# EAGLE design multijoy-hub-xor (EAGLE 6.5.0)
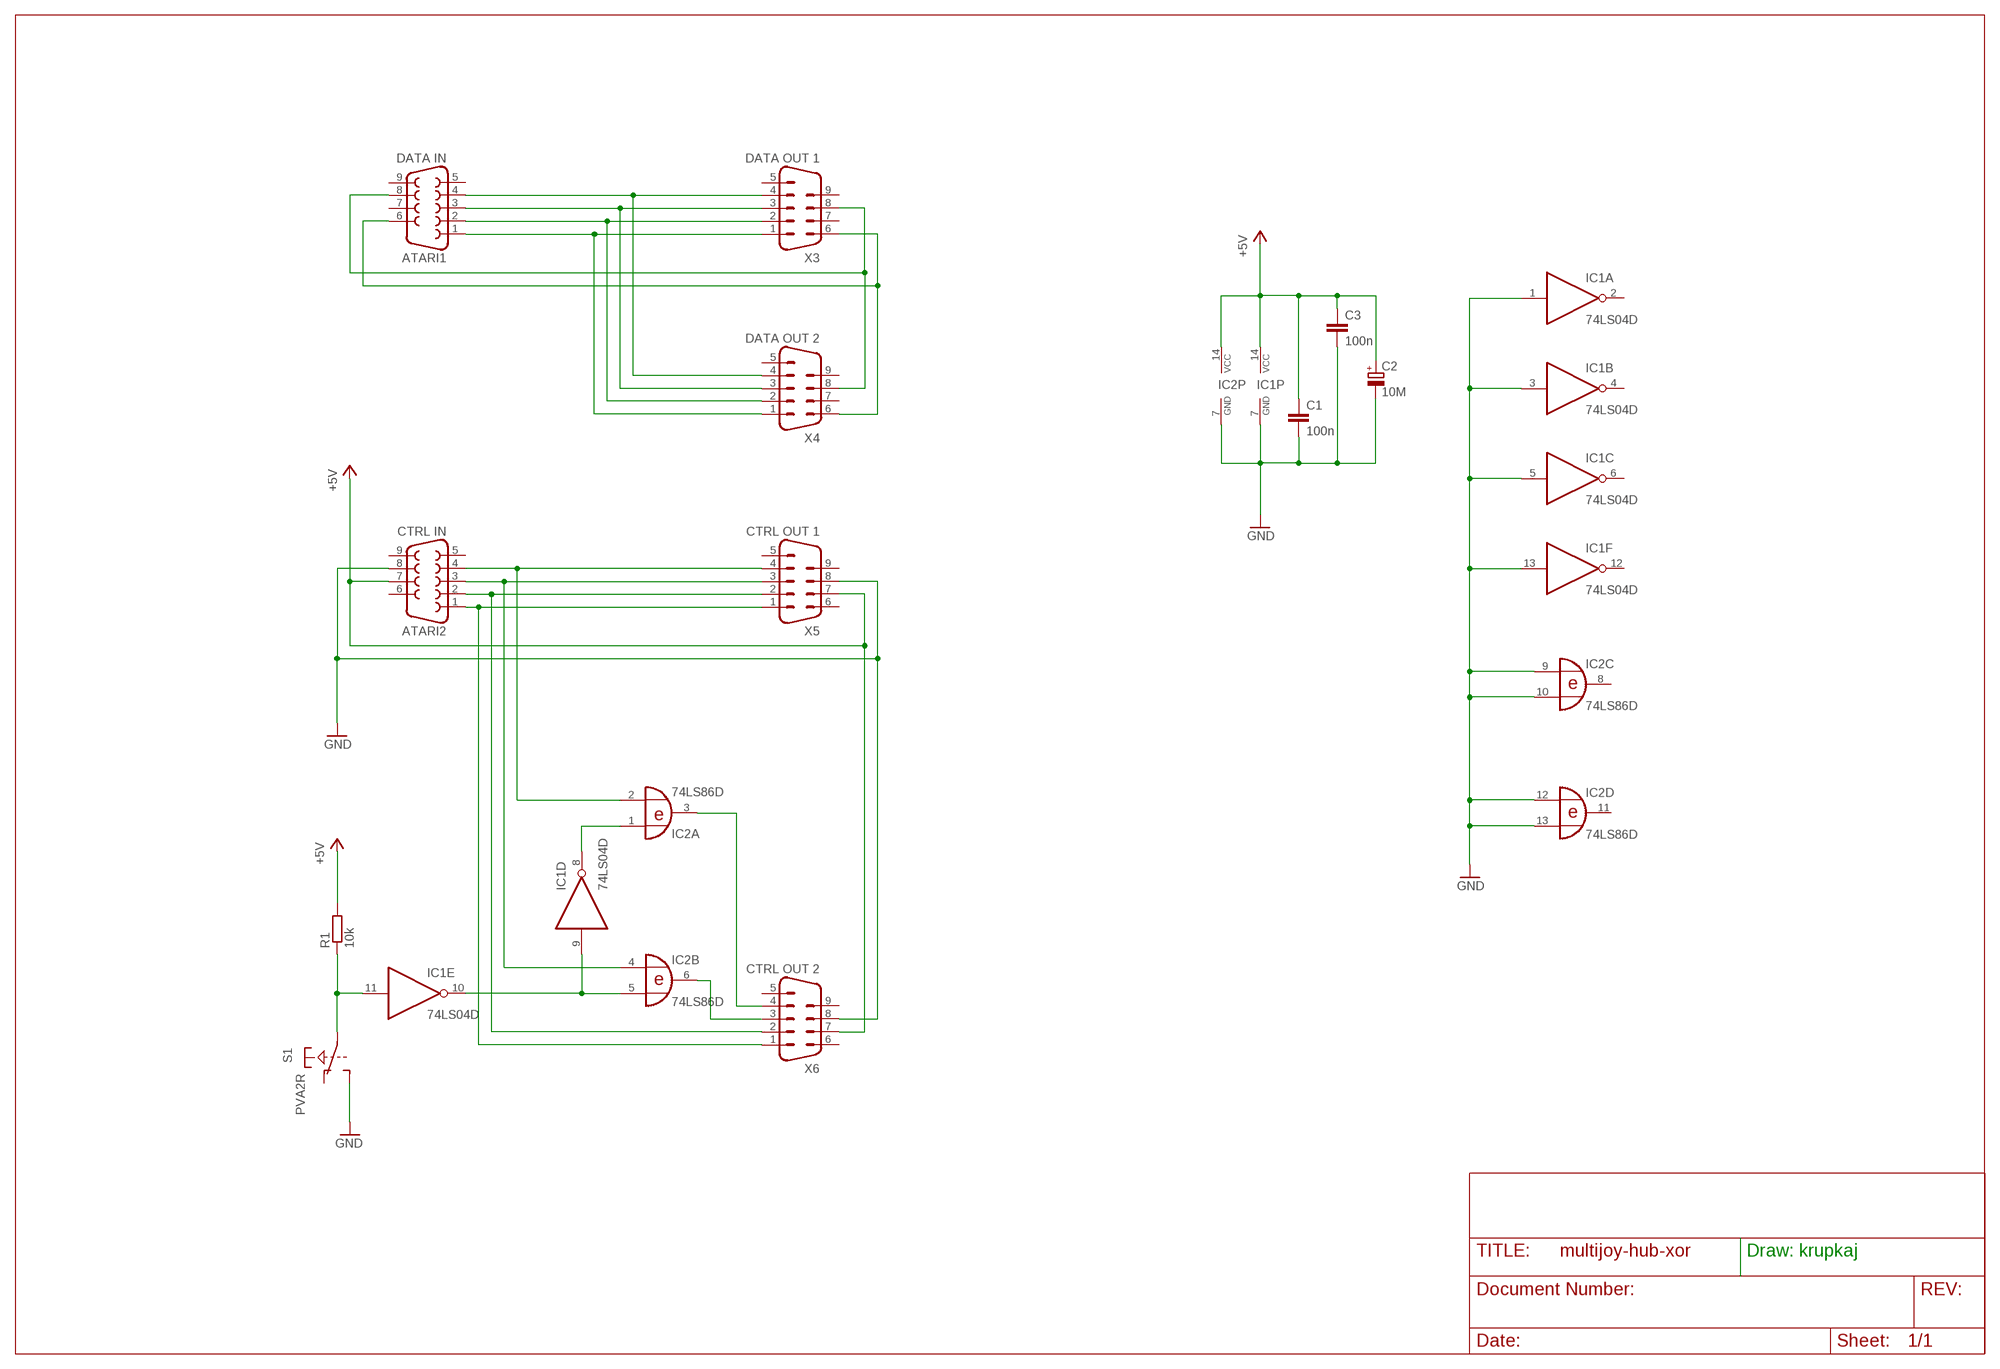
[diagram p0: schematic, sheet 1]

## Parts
ATARI1  DATA IN  F09HP  [F09HP]
ATARI2  CTRL IN  F09HP  [F09HP]
C1  100n  C-EUC0805  [C0805]
C2  10M  CPOL-EUE2.5-6  [E2,5-6]
C3  100n  C-EUC0805  [C0805]
IC1  74LS04D  [SO14]
IC2  74LS86D  [SO14]
R1  10k  R-EU_R0805  [R0805]
S1  PVA2R  [PVA2R]
X3  DATA OUT 1  M09HP  [M09HP]
X4  DATA OUT 2  M09HP  [M09HP]
X5  CTRL OUT 1  M09HP  [M09HP]
X6  CTRL OUT 2  M09HP  [M09HP]

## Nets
+5V: ATARI2.7 C1.1 C2.+ C3.1 IC1.14(P:VCC) IC2.14(P:VCC) R1.2 X5.7 X6.7
GND: ATARI2.8 C1.2 C2.- C3.2 IC1.1(A:I) IC1.3(B:I) IC1.5(C:I) IC1.7(P:GND) IC1.13(F:I) IC2.7(P:GND) IC2.9(C:I0) IC2.10(C:I1) IC2.12(D:I0) IC2.13(D:I1) S1.1(1:S) X5.8 X6.8
N$1: ATARI1.1 X3.1 X4.1
N$2: ATARI1.2 X3.2 X4.2
N$3: ATARI1.3 X3.3 X4.3
N$4: ATARI1.4 X3.4 X4.4
N$5: ATARI2.1 X5.1 X6.1
N$6: ATARI2.2 X5.2 X6.2
N$7: ATARI1.6 X3.6 X4.6
N$8: IC2.6(B:O) X6.3
N$9: ATARI2.3 IC2.4(B:I0) X5.3
N$10: ATARI2.4 IC2.2(A:I1) X5.4
N$11: IC2.3(A:O) X6.4
N$12: IC1.9(D:I) IC1.10(E:O) IC2.5(B:I1)
N$13: IC1.8(D:O) IC2.1(A:I0)
N$14: ATARI1.8 X3.8 X4.8
N$18: IC1.11(E:I) R1.1 S1.2(1:P)
Unconnected: ATARI1.5 ATARI1.7 ATARI1.9 ATARI2.5 ATARI2.6 ATARI2.9 IC1.2(A:O) IC1.4(B:O) IC1.6(C:O) IC1.12(F:O) IC2.8(C:O) IC2.11(D:O) S1.3(1:O) S1.4(2:S) S1.5(2:P) S1.6(2:O) X3.5 X3.7 X3.9 X4.5 X4.7 X4.9 X5.5 X5.6 X5.9 X6.5 X6.6 X6.9

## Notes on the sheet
- Draw: krupkaj

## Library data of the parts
ATARI1 ATARI2 = con-subd:F09: SUB-D
C1 C3 = rcl:C-EU: CAPACITOR, European symbol
C2 = rcl:CPOL-EU: POLARIZED CAPACITOR, European symbol
IC1 = 74xx-eu:74*04: Hex INVERTER
IC2 = 74xx-eu:74*86: Quad 2-input EXCLUSIVE-OR (XOR) gate
R1 = rcl:R-EU_: RESISTOR, European symbol
S1 = switch-misc:PVA2R: ITT SWITCH
X3-X6 = con-subd:M09: SUB-D

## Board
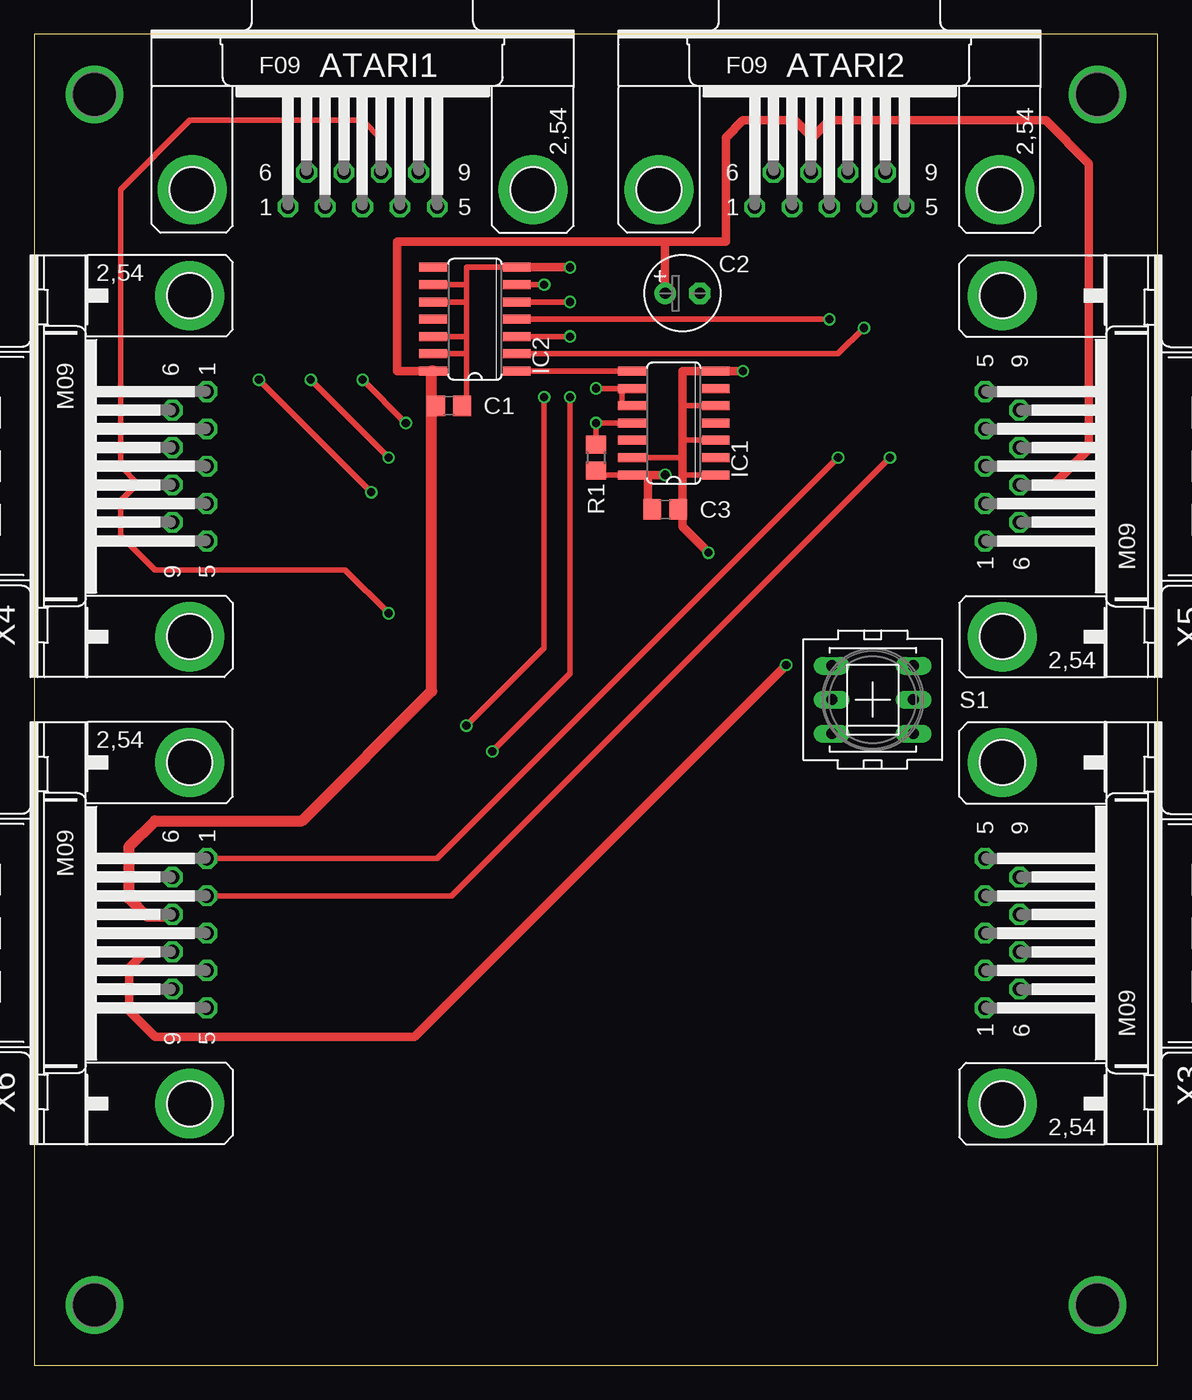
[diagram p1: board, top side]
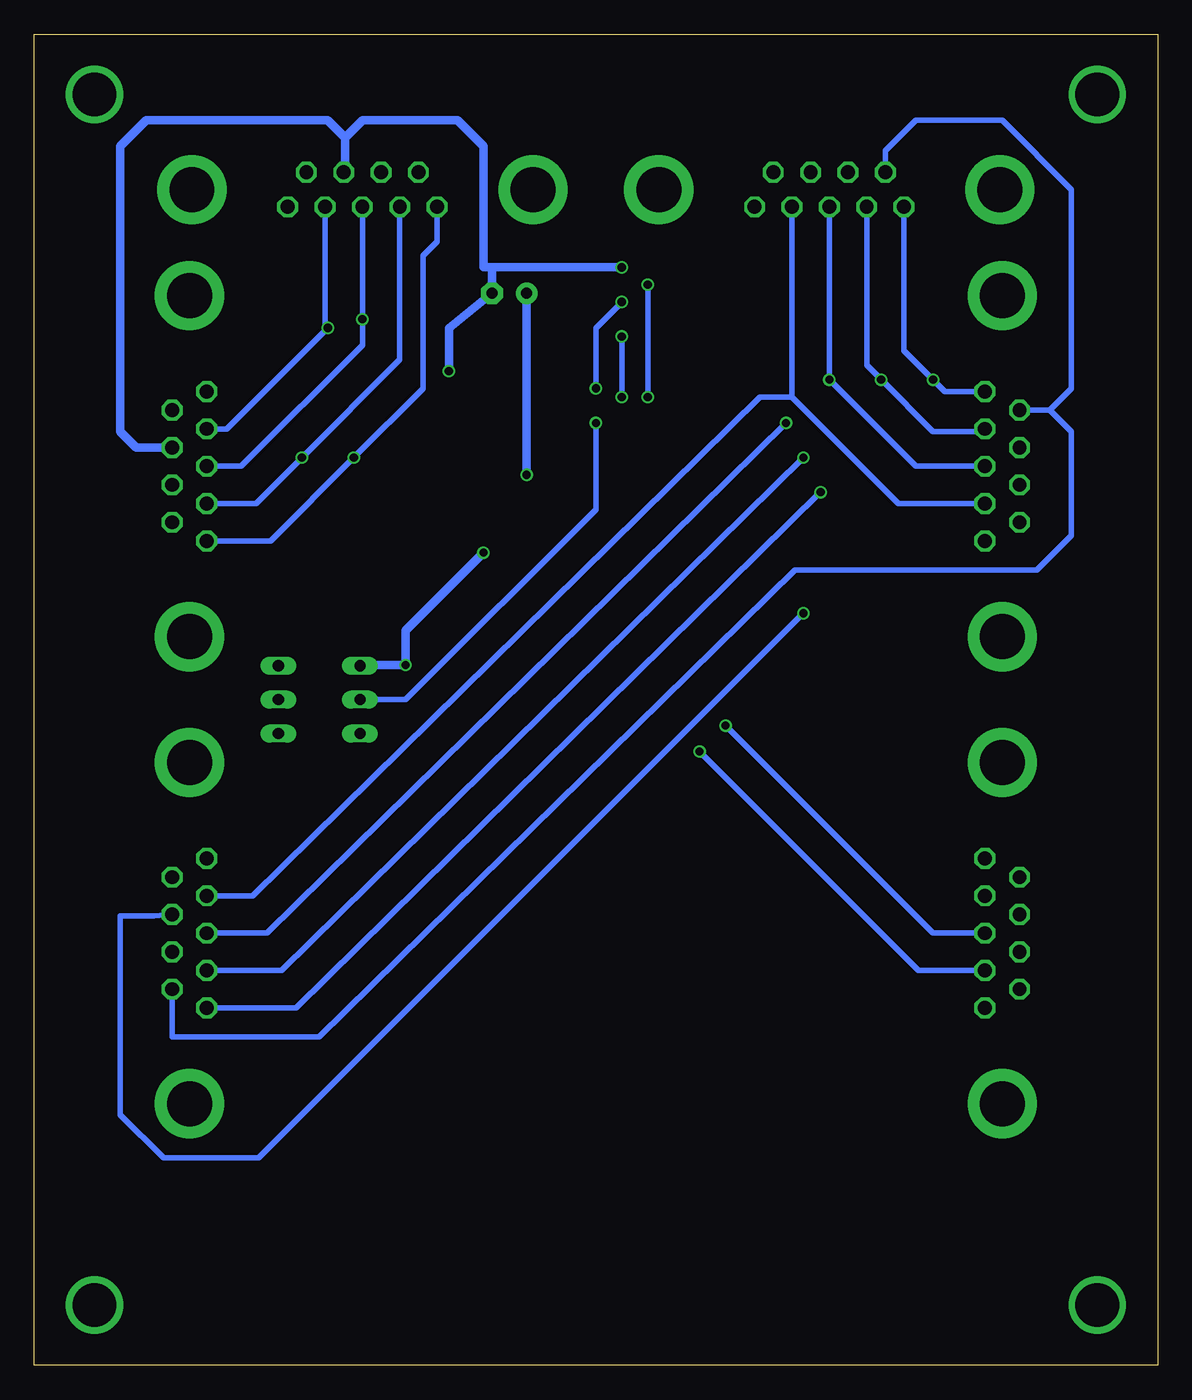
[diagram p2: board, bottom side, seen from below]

Size 82.54 x 97.78 mm. Coordinates in mm from the lower left corner, seen from the top.
Outline: 0,0 82.54,0 82.54,97.78 0,97.78 0,0
Copper layers (1*16): Top 0.035mm / dielectric 1.5mm / Bottom 0.035mm
Design rules "SeeedStudio_2layer_DRU_no_angle_20140221": minimum track width 6mil, minimum drill 12mil, track to track 6mil, track to pad 6mil, pad to pad 6mil, via to via 6mil, smd to smd 0mil, copper to edge 10mil, drill to drill 10mil, minimum pad ring 10mil, minimum via ring 6mil, stop-mask expansion 2mil, vias tented up to drill 100mil, thermal gap 10mil

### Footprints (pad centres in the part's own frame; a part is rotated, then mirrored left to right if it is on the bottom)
F09HP = drill 1.016 octagon: 1 -5.486,-1.27; 2 -2.743,-1.27; 3 0,-1.27; 4 2.743,-1.27; 5 5.486,-1.27; 6 -4.115,1.27; 7 -1.372,1.27; 8 1.372,1.27; 9 4.115,1.27 | drill 3.302 pad 5.08: G1 -12.522,0; G2 12.522,0
C0805 = smd 1.3 x 1.5: 1 -0.95,0; 2 0.95,0
E2,5-6 = drill 0.813 pad 1.6: + -1.27,0 | drill 0.813 pad 1.6 octagon: - 1.27,0
SO14 = smd 0.66 x 2.032: 1 -3.81,-3.073; 2 -2.54,-3.073; 3 -1.27,-3.073; 4 0,-3.073; 5 1.27,-3.073; 6 2.54,-3.073; 7 3.81,-3.073; 8 3.81,3.073; 9 2.54,3.073; 10 1.27,3.073; 11 0,3.073; 12 -1.27,3.073; 13 -2.54,3.073; 14 -3.81,3.073
R0805 = smd 1.3 x 1.5: 1 -0.95,0; 2 0.95,0
PVA2R = drill 0.813 long: 1 -2.997,2.489; 2 -2.997,0; 3 -2.997,-2.489; 4 2.997,2.489; 5 2.997,0; 6 2.997,-2.489
M09HP = drill 1.016 octagon: 1 -5.486,1.27; 2 -2.743,1.27; 3 0,1.27; 4 2.743,1.27; 5 5.486,1.27; 6 -4.115,-1.27; 7 -1.372,-1.27; 8 1.372,-1.27; 9 4.115,-1.27 | drill 3.302 pad 5.08: G1 -12.522,0; G2 12.522,0

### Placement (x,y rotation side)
ATARI1  24.13,86.36 0 top
ATARI2  58.42,86.36 0 top
C1  30.48,70.48 0 top
C2  47.62,78.74 0 top
C3  46.35,62.86 0 top
IC1  46.99,69.22 90 top
IC2  32.38,76.84 90 top
R1  41.27,66.67 270 top
S1  61.59,48.89 0 top
X3  71.12,31.75 90 top
X4  11.43,66.04 270 top
X5  71.12,66.04 90 top
X6  11.43,31.75 270 top

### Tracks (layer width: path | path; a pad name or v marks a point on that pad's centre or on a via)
+5V  (via drill 0.6)
  Top 0.406: 57.15,90.17 57.15,87.73 ATARI2.7 57.05,90.27 | IC2.14 29.84,73.03 | 29.84,73.03 30.35,73.03 | 10.16,33.02 X6.7 | 29.21,73.03 29.58,73.03 29.71,72.89 29.84,73.03 | 45.09,65.28 44.95,65.41 IC1.14 | 29.21,70.48 C1.1 | C3.1 45.09,62.86 | 45.09,65.41 41.27,65.41 R1.2
  Top 0.61: X5.7 74.83,64.67 77.47,67.31 77.47,88.27 74.3,91.44 58.42,91.44 57.15,90.17 | 57.05,90.27 55.88,91.44 52.07,91.44 50.8,90.17 50.8,82.55 46.35,82.55 | 45.09,65.41 45.09,65.28 45.09,62.86 | 46.35,82.55 C2.+ | 46.35,82.55 26.67,82.55 26.67,73.03 29.21,73.03 | v46.35,65.41 45.09,65.41 | 45.09,65.41 IC1.14
  Top 0.813: 10.16,33.02 8.26,33.02 6.99,34.29 6.99,38.1 8.89,40 19.68,40 29.21,49.53 29.21,70.48 29.21,73.03 IC2.14
  Bottom 0.61: C2.+ v46.35,65.41
GND  (via drill 0.6)
  Top 0.406: 47.62,62.23 47.62,62.86 | C1.2 31.75,70.48 31.75,74.3 | 31.75,74.3 IC2.13 | 31.75,75.56 IC2.12 | 31.75,75.56 31.75,74.3 | 31.75,79.38 IC2.9 | 31.75,78.11 31.75,75.56 | 31.75,79.38 31.75,78.11 | 31.75,78.11 IC2.10 | 31.75,79.38 31.75,80.64 IC2.7 | 47.62,70.48 IC1.5 | 47.62,65.41 IC1.1 | 47.62,67.94 IC1.3 | 47.62,66.67 IC1.13
  Top 0.61: v52.07,73.03 IC1.7 47.62,73.03 47.62,70.48 47.62,67.94 47.62,66.67 47.62,65.41 47.62,62.86 C3.2 46.99,62.86 | v39.37,80.64 IC2.7 | v49.53,59.69 47.62,61.59 47.62,62.23 | X6.8 8.15,30.38 6.99,29.21 6.99,26.04 8.89,24.13 27.94,24.13 v55.24,51.44
  Bottom 0.406: 59.69,87.73 ATARI2.8
  Bottom 0.61: 48.89,80.64 C2.- 52.07,76.2 v52.07,73.03 | 48.89,80.64 49.53,80.64 49.53,89.53 51.44,91.44 58.42,91.44 59.69,90.17 | 59.69,90.17 59.69,87.73 | X5.8 75.03,67.41 76.2,68.58 76.2,89.53 74.3,91.44 60.96,91.44 59.69,90.17 | 48.89,80.64 v39.37,80.64 | v49.53,59.69 55.24,53.97 v55.24,51.44 58.55,51.44 S1.1
N$1  (via drill 0.6)
  Top 0.406: v16.51,72.39 v24.77,64.14
  Bottom 0.406: X4.1 15.65,71.53 v16.51,72.39 18.64,74.52 ATARI1.1 | X3.1 63.27,26.26 v24.77,64.14
N$2  (via drill 0.6)
  Top 0.406: v20.32,72.39 v26.04,66.67
  Bottom 0.406: ATARI1.2 21.39,73.46 v20.32,72.39 16.51,68.58 12.9,68.58 X4.2 | X3.2 64.34,29.01 v26.04,66.67
N$3  (via drill 0.6)
  Top 0.406: v24.13,72.39 v27.3,69.22
  Bottom 0.406: ATARI1.3 v24.13,72.39 17.78,66.04 X4.3 | X3.3 65.41,31.75 v27.3,69.22
N$4
  Bottom 0.406: X4.4 19.05,63.3 26.87,71.12 | X3.4 66.47,34.49 29.21,71.12 26.87,71.12 | 26.87,71.12 ATARI1.4
N$5  (via drill 0.6)
  Top 0.406: X6.1 29.62,37.24 v59.05,66.67
  Bottom 0.406: X5.1 65.18,60.55 v59.05,66.67 53.98,71.75 53.98,81.51 52.93,82.55 ATARI2.1
N$6  (via drill 0.6)
  Top 0.406: X6.2 30.68,34.49 v62.86,66.67
  Bottom 0.406: ATARI2.2 55.68,73.86 v62.86,66.67 66.24,63.3 X5.2
N$7
  Bottom 0.406: ATARI1.6 20.02,89.2 17.78,91.44 11.43,91.44 6.35,86.36 6.35,71.73 7.92,70.16 | X3.6 72.39,24.13 61.59,24.13 26.67,58.42 8.89,58.42 6.35,60.96 6.35,68.58 7.92,70.16 | 7.92,70.16 X4.6
N$8  (via drill 0.6)
  Top 0.406: v31.75,46.99 37.46,52.7 v37.46,71.12 | v37.46,79.38 IC2.6
  Bottom 0.406: X6.3 16.51,31.75 v31.75,46.99 | v37.46,71.12 v37.46,79.38
N$9  (via drill 0.6)
  Top 0.406: IC2.4 v58.42,76.84
  Bottom 0.406: ATARI2.3 v58.42,76.84 58.42,74.93 67.31,66.04 X5.3
N$10  (via drill 0.6)
  Top 0.406: IC2.2 59.05,74.3 v60.96,76.2
  Bottom 0.406: 61.16,76.2 61.16,76 68.38,68.78 X5.4 | 61.16,76.2 ATARI2.4 | v60.96,76.2 61.16,76.2
N$11  (via drill 0.6)
  Top 0.406: v33.66,45.08 39.37,50.8 v39.37,71.12 | v39.37,75.56 IC2.3
  Bottom 0.406: X6.4 17.58,29.01 v33.66,45.08 | v39.37,71.12 v39.37,75.56
N$12  (via drill 0.6)
  Top 0.406: IC1.10 43.18,70.48 43.18,71.75 IC1.9 v41.27,71.75 | v39.37,78.11 IC2.5
  Bottom 0.406: v41.27,71.75 41.27,76.2 v39.37,78.11
N$13
  Top 0.406: IC2.1 IC1.8
N$14  (via drill 0.6)
  Top 0.406: v26.04,55.25 22.86,58.42 8.89,58.42 6.35,60.96 6.35,63.5 7.62,64.77 | X4.8 8.99,64.67 8.89,64.77 7.62,64.77 | ATARI1.8 25.5,90.07 24.13,91.44 11.43,91.44 6.35,86.36 6.35,66.04 7.62,64.77
  Bottom 0.406: v26.04,55.25 66.04,15.24 73.03,15.24 76.2,18.41 76.2,33.02 73.76,33.02 X3.8
N$15  (via drill 3.2)
  other vias: 78.11,93.34
N$16  (via drill 3.2)
  other vias: 78.11,4.44
N$17  (via drill 3.2)
  other vias: 4.44,4.44
N$18  (via drill 0.6)
  Top 0.406: IC1.11 v41.27,69.22 R1.1
  Bottom 0.406: S1.2 55.24,48.89 41.27,62.86 v41.27,69.22
N$19  (via drill 3.2)
  other vias: 4.44,93.34

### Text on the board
tDocu: MultiJoy Hub | krupkaj | 2014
